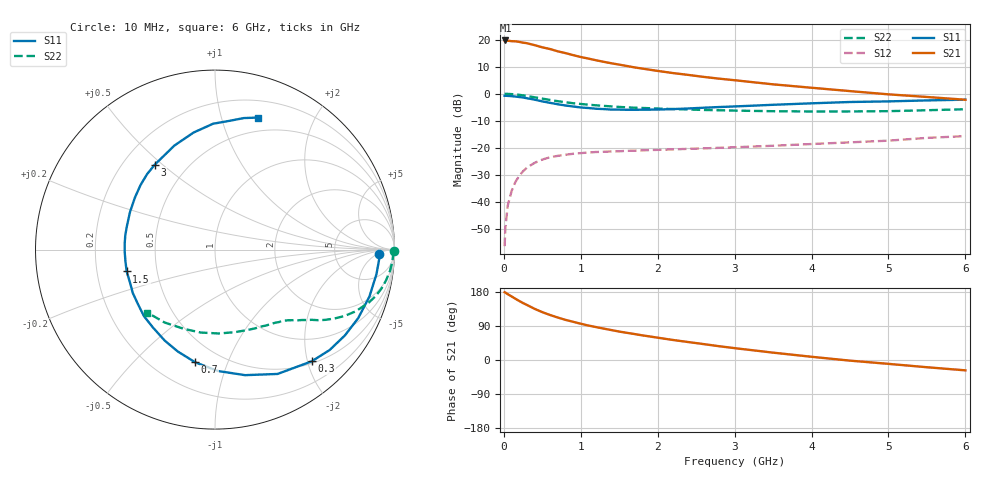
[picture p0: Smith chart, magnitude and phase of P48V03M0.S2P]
! SIEMENS Small Signal Semiconductors
! BFP182
! Si NPN RF Bipolar Junction Transistor in SOT143
! VCE = 8 V  IC = 3 mA
! Common Emitter S-Parameters:  March  1996
# GHz  S  MA  R  50
!  f  S11  S21  S12  S22
! GHz  MAG  ANG  MAG  ANG  MAG  ANG  MAG  ANG
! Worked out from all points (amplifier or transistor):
!   36 points, 10 MHz to 6 GHz, reference 50 ohm
!   highest |S21| = 19.7 dB at 20 MHz (marker M1)
!   |S21| within 3 dB of that: start of sweep to 572.4 MHz
!   unconditionally stable (mu >= 1): 1.989 GHz to 5.89 GHz
!   at 250 MHz: K = 0.16, MSG = 23.8 dB, |S12| = -28.7 dB
!   at 1.4 GHz: K = 0.76, MSG = 16.3 dB, |S12| = -21.4 dB
!   at 6 GHz: K = 0.98, MSG = 6.7 dB, |S12| = -15.7 dB
!   S11 on the Smith chart (normalised r, x): 10 MHz: 20, -6; 300 MHz: 0.54, -2.08; 700 MHz: 0.36, -0.77; 1.5 GHz: 0.33, -0.11; 3 GHz: 0.33, +0.47; 6 GHz: 0.36, +1.32
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0.01  0.9144 -1.6  9.52 178.8  0.0015 80.9  0.9946 -0.6
0.02  0.9159 -3.5  9.672 177.9  0.0033 84.4  0.9932 -1.4
0.05  0.91 -8.6  9.581 173.8  0.0084 84.1  0.991 -3.5
0.15  0.8845 -25.6  9.327 161.7  0.0232 75.3  0.9683 -10.2
0.2  0.8676 -33.4  9.099 155.8  0.0301 71.2  0.9517 -13.3
0.3  0.8233 -49.1  8.604 145.3  0.0426 62.7  0.9061 -19.0
0.4  0.7755 -63.3  7.919 135.0  0.0524 56.0  0.8571 -23.6
0.5  0.7194 -76.5  7.221 126.3  0.0602 50.0  0.8103 -27.2
0.6  0.6769 -88.5  6.71 118.8  0.0665 45.0  0.7664 -30.1
0.7  0.6374 -100.0  6.089 112.1  0.0705 41.0  0.7269 -32.6
0.8  0.6043 -110.1  5.647 106.0  0.074 37.5  0.6941 -34.5
0.9  0.5793 -118.9  5.176 100.8  0.0771 35.2  0.6656 -36.0
1.1  0.5424 -136.9  4.462 90.9  0.0814 30.7  0.6247 -38.9
1.3  0.518 -152.1  3.886 82.8  0.084 27.7  0.5939 -41.4
1.5  0.5069 -166.1  3.45 75.0  0.0858 26.0  0.5685 -43.8
1.8  0.5044 176.0  2.914 65.0  0.0892 24.1  0.5438 -47.3
2.2  0.5181 156.0  2.407 52.8  0.0929 22.8  0.5188 -52.9
3  0.5801 125.3  1.774 31.3  0.1018 22.1  0.4859 -66.4
3.5  0.6224 111.3  1.489 19.4  0.1085 21.4  0.4735 -76.2
4.5  0.7013 90.9  1.116 -1.7  0.1255 19.8  0.4688 -99.6
5.5  0.7504 77.6  0.869 -19.1  0.1518 17.8  0.4937 -124.6
6  0.7743 71.8  0.772 -27.3  0.1638 14.4  0.515 -137.1
